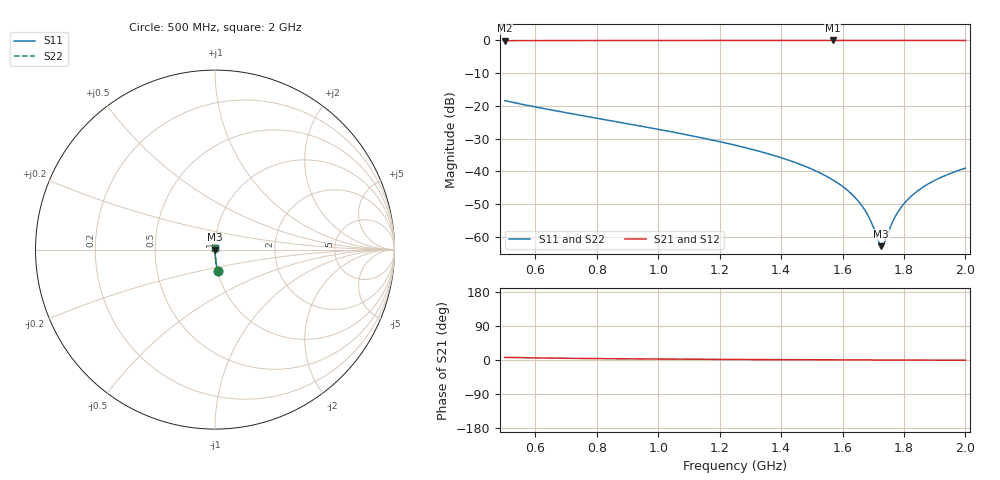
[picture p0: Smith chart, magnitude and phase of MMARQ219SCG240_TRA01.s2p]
! MMARQ219SCG240_TRA01  S-PARAMETER MODEL  ( General Type )
! Model Generated by TAIYO YUDEN Corporation (http://www.ty-top.com)
! Version 1.0
! TAIYO YUDEN Control No. 180601
! Copyright(c) 2018 TAIYO YUDEN CO.,LTD. All Rights Reserved.
! Product Description (link to TY-COMPAS)
! https://ds.yuden.co.jp/TYCOMPAS/or/detail?pn=MMARQ219SCG240JTRA01&u=M
! Products Name : Multilayer Ceramic Capacitors
! Characteristics :
!  Capacitance : 24 pF , Rated Voltage : 250V , TCC : CG / C0G
!  Case Size : 2.0 x 1.25 / 0.079 x 0.049 [mm/inch] , Thickness : 0.85 / 0.033 [mm/inch]
!  (Conditions: Temperature = 25 degC , DC Bias Current/Voltage = 0A / 0V)
! External Node Assignments :
!  1  o---| |---o  2
! GND o---------o GND
! Frequency Range : 500MHz  -  2000MHz  [ 401 STEP ]
# MHz S RI R 50
! Freq[MHz].  S11 Real  S11 Imag  S21 Real  S21 Imag  S12 Real  S12 Imag  S22 Real  S22 Imag
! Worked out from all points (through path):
!   401 points, 500 MHz to 2 GHz, reference 50 ohm
!   highest |S21| = -0.01 dB at 1.569 GHz (marker M1); lowest = -0.1 dB at 500 MHz (marker M2)
!   group delay of S21, straight-line fit = 12.3 ps
!   lowest |S11| = -62.8 dB at 1.726 GHz (marker M3), VSWR 1.00, Z = 50.1 - j0.00678 ohm
!   |S11| at or under -10 dB: start of sweep to end of sweep
!   |S22| runs from -62.8 to -18.4 dB; largest |S21 - S12| = 0
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500  0.0149 -0.1198  0.9851 0.1198  0.9851 0.1198  0.0149 -0.1198
751.25  0.0055 -0.0712  0.9945 0.0712  0.9945 0.0712  0.0055 -0.0712
1002.5  0.00239 -0.0437  0.9976 0.0437  0.9976 0.0437  0.00239 -0.0437
1250  0.00119 -0.0252  0.9988 0.0252  0.9988 0.0252  0.00119 -0.0252
1392.5  0.00088 -0.0166  0.9991 0.0166  0.9991 0.0166  0.00088 -0.0166
1501.25  0.000758 -0.0108  0.9992 0.0108  0.9992 0.0108  0.000758 -0.0108
1568.75  0.00072 -0.00739  0.9993 0.00739  0.9993 0.00739  0.00072 -0.00739
1621.25  0.000708 -0.00487  0.9993 0.00487  0.9993 0.00487  0.000708 -0.00487
1658.75  0.000707 -0.00312  0.9993 0.00312  0.9993 0.00312  0.000707 -0.00312
1685  0.000711 -0.00192  0.9993 0.00192  0.9993 0.00192  0.000711 -0.00192
1696.25  0.000713 -0.00141  0.9993 0.00141  0.9993 0.00141  0.000713 -0.00141
1718.75  0.000719 -0.0004  0.9993 0.0004  0.9993 0.0004  0.000719 -0.0004
1726.25  0.000722 -6.77e-05  0.9993 6.77e-05  0.9993 6.77e-05  0.000722 -6.77e-05
1730  0.000723 9.81e-05  0.9993 -9.81e-05  0.9993 -9.81e-05  0.000723 9.81e-05
1737.5  0.000726 0.000429  0.9993 -0.000429  0.9993 -0.000429  0.000726 0.000429
1752.5  0.000733 0.00109  0.9993 -0.00109  0.9993 -0.00109  0.000733 0.00109
1771.25  0.000742 0.0019  0.9993 -0.0019  0.9993 -0.0019  0.000742 0.0019
1790  0.000752 0.0027  0.9992 -0.0027  0.9992 -0.0027  0.000752 0.0027
1812.5  0.000766 0.00366  0.9992 -0.00366  0.9992 -0.00366  0.000766 0.00366
1838.75  0.000785 0.00476  0.9992 -0.00476  0.9992 -0.00476  0.000785 0.00476
1910  0.000847 0.00767  0.9992 -0.00767  0.9992 -0.00767  0.000847 0.00767
2000  0.000946 0.0112  0.9991 -0.0112  0.9991 -0.0112  0.000946 0.0112
